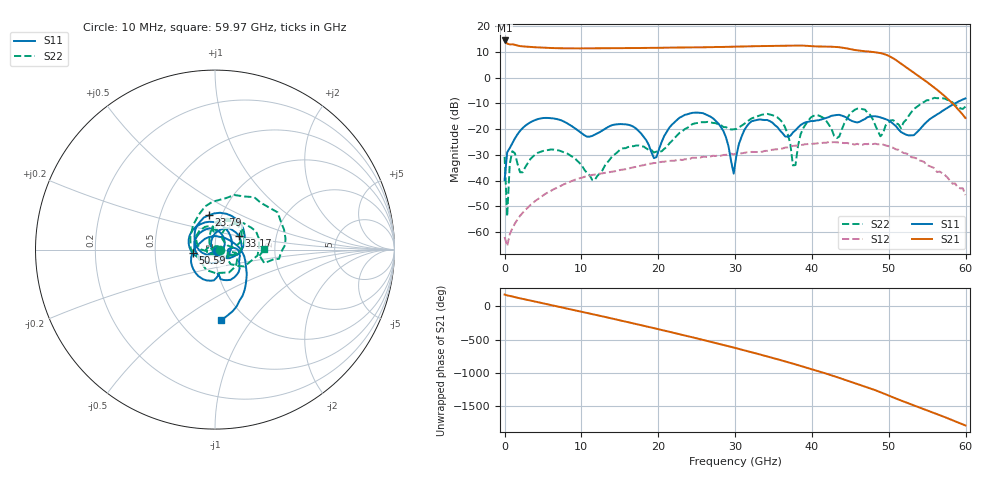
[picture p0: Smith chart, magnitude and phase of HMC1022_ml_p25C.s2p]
! Hittite Microwave Corporation
! 20 Alpha Road
! Chelmsford, MA 01824
! http://www.hittite.com
! Tel: 978-250-3343
! Fax: 978-250-3373
! Device:  HMC1022
! Description: GaAs pHEMT MMIC 0.25 Watt Power Amplifier
! Frequency:  DC -  48.00 GHz
! Package:  DIE
! Ports:  2 RF, 6 DC
!  Pad 1 = RF In  = Port 1
!  Pad 2 = Vg2
!  Pad 3 = ACG1
!  Pad 4 = ACG2
!  Pad 5 = RF Out & Vdd = Port 2
!  Pad 6 = ACG3
!  Pad 7 = ACG4
!  Pad 8 = Vg1
! Voltages:  Vdd =  10.000 Volts,  Idd = 151.40 mA
!  Vg2 =  4.500 Volts,  Idd =  4.20 uA
!  Vdd =  -0.332 Volts,  Idd =  -0.38 mA
! Data:  The device was measured using G-S-G Probes with a microstrip
!  launch (0.25 inch) and two wire bonds to the die.  The reference plane
!  is at the microstrip launch.
!  Data was collected using an calibrated network analyzer.
! Misc:  VU1,  +25 C
! Date Measured:  2011-08-31
! Date:  2012-08-02 MJV
! Note:
!  Hittite supplies this data as a sample of measured data at the package pin for
!  for this package product.  Your particular data for this product may vary.
!  Data was taken at 25 degrees C.
!  Hittite reserves the right to change this data at anytime.
!Freq	S11mag	S11ph	S21mag	S21ph	S12mag	S12ph	S22mag	S22ph
# GHZ S DB R 50.0
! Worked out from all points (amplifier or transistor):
!   180 points, 10 MHz to 59.97 GHz, reference 50 ohm
!   highest |S21| = 14.4 dB at 10 MHz (marker M1)
!   |S21| within 3 dB of that: 12.99 GHz to 44.38 GHz (31.39 GHz wide, 109 % of centre)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
!   unconditionally stable (mu >= 1): start of sweep to end of sweep
!   at 10.06 GHz: K = 11.78, MAG = 11.4 dB, |S12| = -38.9 dB
!   at 30.16 GHz: K = 3.74, MAG = 12.1 dB, |S12| = -29.5 dB
!   at 59.97 GHz: K = 452.08, MAG = -14.6 dB, |S12| = -45.6 dB
!   S11 on the Smith chart (normalised r, x): 10 MHz: 1.02, -0.01; 23.79 GHz: 0.87, +0.35; 33.17 GHz: 1.29, +0.20; 50.59 GHz: 0.78, -0.03; 59.97 GHz: 0.78, -0.72
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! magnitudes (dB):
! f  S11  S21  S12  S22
! 10 MHz  -39.8  14.4  -61.9  -30.8
! 344.9 MHz  -29.0  13.2  -65.5  -53.9
! 679.9 MHz  -27.3  12.9  -60.9  -33.5
! 1.015 GHz  -25.5  12.9  -58.5  -28.6
! 2.355 GHz  -19.6  12.1  -52.5  -36.8
! 5.034 GHz  -15.7  11.6  -45.7  -28.5
! 10.06 GHz  -21.7  11.4  -38.9  -34.1
! 20.11 GHz  -27.7  11.6  -32.9  -28.7
! 23.79 GHz  -14.2  11.8  -31.7  -19.5
! 27.81 GHz  -17.7  11.9  -30.2  -18.2
! 29.82 GHz  -37.3  12.0  -29.8  -20.1
! 30.16 GHz  -30.5  12.1  -29.5  -20.0
! 33.17 GHz  -16.2  12.2  -28.9  -14.7
! 36.18 GHz  -21.6  12.4  -27.5  -17.4
! 37.52 GHz  -21.3  12.5  -26.5  -34.1
! 40.2 GHz  -16.9  12.2  -25.6  -14.9
! 43.22 GHz  -14.5  11.9  -25.1  -23.5
! 45.9 GHz  -17.4  10.6  -25.7  -12.0
! 48.91 GHz  -15.4  9.5  -25.9  -22.8
! 50.25 GHz  -17.1  8.0  -27.0  -16.6
! 50.59 GHz  -18.0  7.5  -27.3  -16.5
! 59.97 GHz  -8.1  -15.7  -45.6  -11.2
